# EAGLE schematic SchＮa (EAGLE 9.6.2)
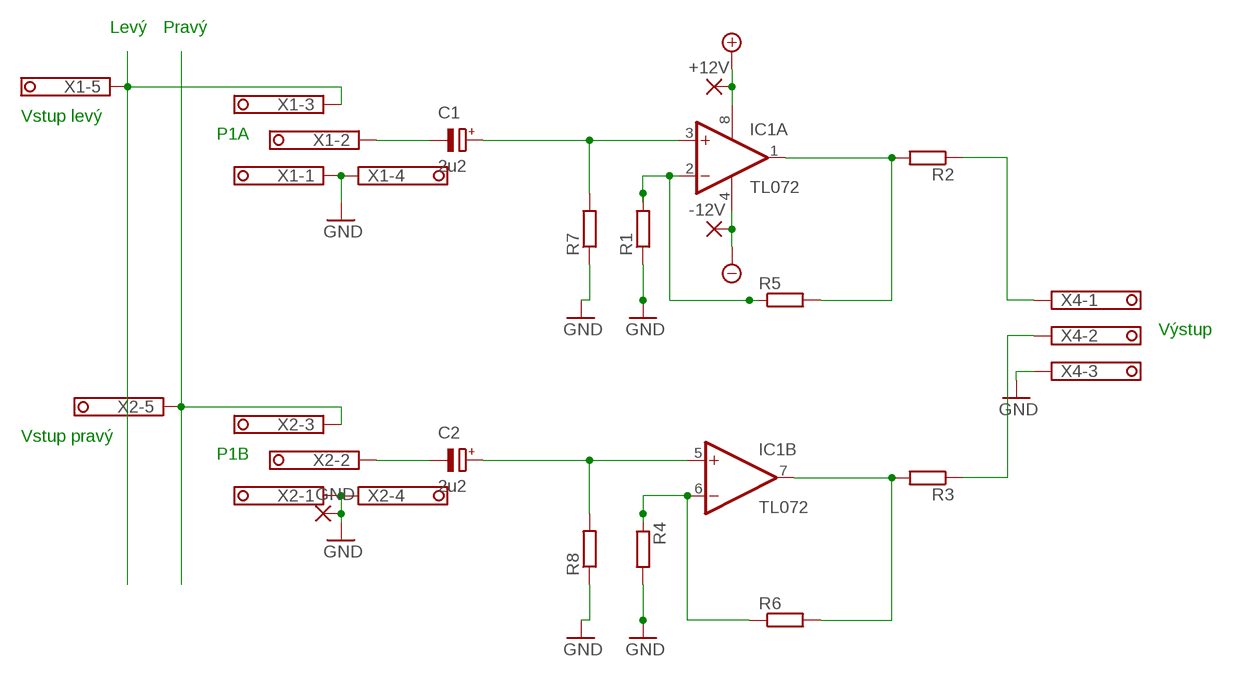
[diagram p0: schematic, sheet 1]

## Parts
+12V  1,6/0,8  [1,6/0,8]
-12V  1,6/0,8  [1,6/0,8]
C1  2u2  CPOL-EUE2,5-6E  [E2,5-6E]
C2  2u2  CPOL-EUE2,5-6E  [E2,5-6E]
GND  1,6/0,8  [1,6/0,8]
IC1  TL072  TL072P  [DIL08]
R1  R-EU_M1206  [M1206]
R2  R-EU_M1206  [M1206]
R3  R-EU_M1206  [M1206]
R4  R-EU_M1206  [M1206]
R5  R-EU_M1206  [M1206]
R6  R-EU_M1206  [M1206]
R7  R-EU_M1206  [M1206]
R8  R-EU_M1206  [M1206]
X1  1751277  [1751277]
X2  1751277  [1751277]
X4  1751251  [1751251]

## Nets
+12V: +12V.1(P) IC1.8(P:V+)
-12V: -12V.1(P) IC1.4(P:V-)
GND: GND.1(P) R1.1 R4.2 R7.1 R8.1 X1.1 X1.4 X2.1 X2.4 X4.3
N$1: C2.- X2.2
N$2: C1.- X1.2
N$3: C1.+ IC1.3(A:+IN) R7.2
N$4: C2.+ IC1.5(B:+IN) R8.2
N$5: IC1.2(A:-IN) R1.2 R5.1
N$6: IC1.1(A:OUT) R2.2 R5.2
N$7: IC1.7(B:OUT) R3.2 R6.2
N$8: IC1.6(B:-IN) R4.1 R6.1
N$9: R3.1 X4.2
N$10: R2.1 X4.1
N$11: X2.3 X2.5
N$12: X1.3 X1.5

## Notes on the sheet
- Levý | Pravý
- Vstup levý
- P1A
- Výstup
- Vstup pravý
- P1B

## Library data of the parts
+12V -12V GND = wirepad:1,6/0,8: THROUGH-HOLE PAD
C1 C2 = rcl:CPOL-EU: POLARIZED CAPACITOR, European symbol; SPICEPREFIX: C
IC1 = linear:TL072: OP AMP
R1-R8 = rcl:R-EU_: RESISTOR, European symbol; SPICEPREFIX: R
X1 X2 = con-phoenix-350:1751277: MKDS 1/ 5-3,5 Printklemme Nennstrom: 10 A Bemessungsspannung: 160 V Raster: 3,5 mm Polzahl: 5 Montageart: Löten Anschlussart: Schraubanschluss Anschlussrichtung vom Leiter zur Platine: 0° Source: http://eshop.phoenixcontact.com .. 1751277.pdf; OC_FARNELL: unknown; OC_NEWARK: unknown
X4 = con-phoenix-350:1751251: MKDS 1/ 3-3,5 Printklemme Nennstrom: 10 A Bemessungsspannung: 160 V Raster: 3,5 mm Polzahl: 3 Montageart: Löten Anschlussart: Schraubanschluss Anschlussrichtung vom Leiter zur Platine: 0° Source: http://eshop.phoenixcontact.com .. 1751251.pdf; OC_FARNELL: unknown; OC_NEWARK: unknown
